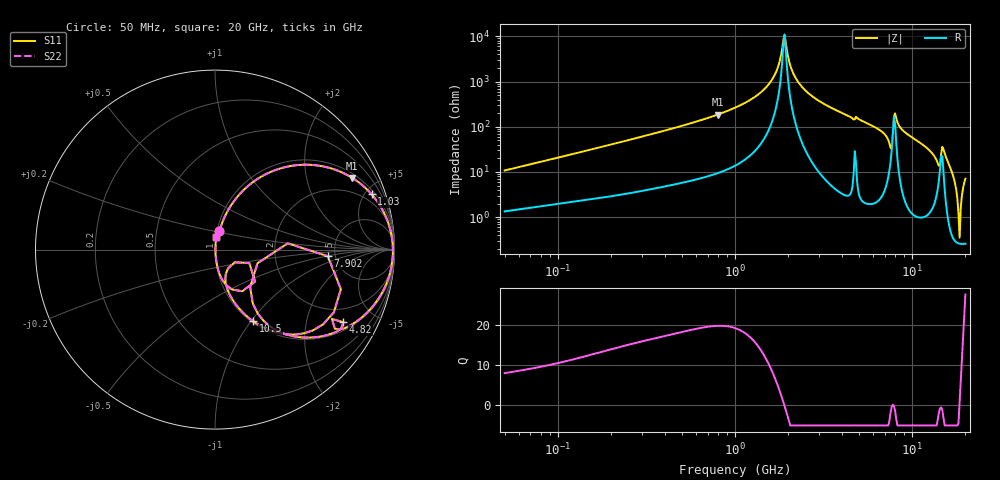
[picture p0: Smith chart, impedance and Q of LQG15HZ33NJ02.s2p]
!Murata Part Number: LQG15HZ33NJ02
!These Parameters are Measured in Series Mode Connection
!  o--[Z]--o
!Port1  Port2
!  o-------o
!Freq. Start=50[MHz] Stop=20[GHz], 401[Steps]
# Hz S RI R 50
!Freq.(Hz) S11(Real) S11(Imag) S21(Real) S21(Imag) S12(Real) S12(Imag) S22(Real) S22(Imag)
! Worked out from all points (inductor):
!   401 points, 50 MHz to 20 GHz, reference 50 ohm
!   read as one part in series: L = 33.5 nH near 51.52 MHz
!   highest Q = 19.7 at 798.8 MHz (marker M1), where L = 37 nH
!   self-resonance near 1.876 GHz
!   S11 on the Smith chart (normalised r, x): 50 MHz: 1.03, +0.21; 1.03 GHz: 1.29, +5.55; 4.82 GHz: 1.32, -3.31; 7.902 GHz: 4.34, -0.53; 10.5 GHz: 1.02, -1.02; 20 GHz: 1.01, +0.14
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5e7  0.0241 0.1029  0.9759 -0.1029  0.9759 -0.1029  0.0241 0.1029
1.364002e8  0.0898 0.2471  0.9102 -0.2471  0.9102 -0.2471  0.0898 0.2471
3.721004e8  0.3728 0.4548  0.6272 -0.4548  0.6272 -0.4548  0.3728 0.4548
7.987718e8  0.7645 0.3997  0.2355 -0.3997  0.2355 -0.3997  0.7645 0.3997
1e9  0.8617 0.3202  0.1383 -0.3202  0.1383 -0.3202  0.8617 0.3202
1.030411e9  0.8729 0.3078  0.1271 -0.3078  0.1271 -0.3078  0.8729 0.3078
1.567309e9  0.9779 0.1047  0.0221 -0.1047  0.0221 -0.1047  0.9779 0.1047
1.904239e9  0.991 -0.00105  0.00895 0.00105  0.00895 0.00105  0.991 -0.00105
2.179053e9  0.9861 -0.0758  0.0139 0.0758  0.0139 0.0758  0.9861 -0.0758
2.728004e9  0.9509 -0.1997  0.0491 0.1997  0.0491 0.1997  0.9509 -0.1997
4.81993e9  0.7154 -0.4049  0.2846 0.4049  0.2846 0.4049  0.7154 -0.4049
6.601595e9  0.4119 -0.4771  0.5881 0.4771  0.5881 0.4771  0.4119 -0.4771
7.442007e9  0.2105 -0.3003  0.7895 0.3003  0.7895 0.3003  0.2105 -0.3003
7.901521e9  0.6288 -0.037  0.3712 0.037  0.3712 0.037  0.6288 -0.037
8.516016e9  0.5005 -0.4653  0.4995 0.4653  0.4995 0.4653  0.5005 -0.4653
1.050288e10  0.2121 -0.3988  0.7879 0.3988  0.7879 0.3988  0.2121 -0.3988
1.396067e10  0.0602 -0.1362  0.9398 0.1362  0.9398 0.1362  0.0602 -0.1362
1.527346e10  0.0949 -0.2219  0.9051 0.2219  0.9051 0.2219  0.0949 -0.2219
1.721783e10  0.00816 -0.0703  0.9918 0.0703  0.9918 0.0703  0.00816 -0.0703
1.800918e10  0.00336 -0.026  0.9966 0.026  0.9966 0.026  0.00336 -0.026
1.855685e10  0.00258 0.00237  0.9974 -0.00237  0.9974 -0.00237  0.00258 0.00237
2e10  0.00755 0.0703  0.9924 -0.0703  0.9924 -0.0703  0.00755 0.0703
